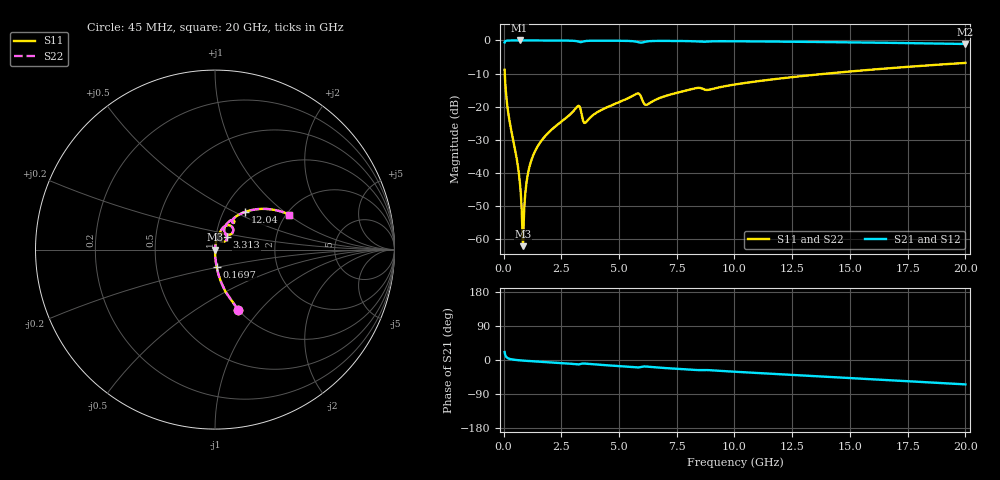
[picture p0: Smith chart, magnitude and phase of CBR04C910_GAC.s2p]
! S-parameter model data by Modelithics Inc.  support@modelithics.com 813-866-6335  Tampa FL USA
! S-Parameter data specifications:
! Substrate: 20-mil Rogers 4350B, substrate thickness, H=0.508mm, Dielectric constant, Er=3.75
! PCB Mounting Pad Footprint: Pad width, PadW=0.52mm , Pad length, PadL=0.52mm , Pad gap, PadG (edge-to-edge)=0.28mm , Reference planes=1.32mm apart
#  GHz  S  MA  R 50
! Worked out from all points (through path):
!   801 points, 45 MHz to 20 GHz, reference 50 ohm
!   highest |S21| = -0.01 dB at 693.5 MHz (marker M1); lowest = -1.1 dB at 20 GHz (marker M2)
!   group delay of S21, straight-line fit = 9.07 ps
!   lowest |S11| = -62.0 dB at 843.2 MHz (marker M3), VSWR 1.00, Z = 50.1 + j0.0259 ohm
!   |S11| at or under -10 dB: 53.06 MHz to 14 GHz (13.95 GHz wide, 198 % of centre)
!   |S22| runs from -62.0 to -6.8 dB; largest |S21 - S12| = 0
!   S11 on the Smith chart (normalised r, x): 45 MHz: 1.00, -0.77; 169.7 MHz: 1.00, -0.20; 3.313 GHz: 1.13, +0.16; 12.04 GHz: 1.26, +0.57; 20 GHz: 2.08, +1.02
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0.045  0.3605 -68.9  0.9326 21.0  0.9326 21.0  0.3605 -68.9
0.169719  0.09807 -84.5  0.9948 5.3  0.9948 5.3  0.09807 -84.5
0.568819  0.01656 -88.0  0.9992 -0.1  0.9992 -0.1  0.01656 -88.0
0.693538  0.007957 -86.0  0.9993 -0.8  0.9993 -0.8  0.007957 -86.0
0.768369  0.003679 -80.2  0.9993 -1.2  0.9993 -1.2  0.003679 -80.2
0.8432  0.000791 19.1  0.9992 -1.6  0.9992 -1.6  0.000791 19.1
0.918031  0.003922 76.7  0.9992 -1.9  0.9992 -1.9  0.003922 76.7
0.992862  0.007208 81.3  0.9991 -2.2  0.9991 -2.2  0.007208 81.3
1.092637  0.01132 83.0  0.9991 -2.7  0.9991 -2.7  0.01132 83.0
1.44185  0.02414 83.6  0.9987 -4.1  0.9987 -4.1  0.02414 83.6
2.115331  0.04629 81.7  0.9975 -6.6  0.9975 -6.6  0.04629 81.7
3.312631  0.09691 46.0  0.9435 -10.8  0.9435 -10.8  0.09691 46.0
3.387462  0.0746 39.5  0.9494 -9.5  0.9494 -9.5  0.0746 39.5
3.562069  0.05821 62.3  0.9804 -9.8  0.9804 -9.8  0.05821 62.3
5.757119  0.1573 59.2  0.9571 -19.5  0.9571 -19.5  0.1573 59.2
6.181163  0.1069 55.8  0.9635 -17.3  0.9635 -17.3  0.1069 55.8
6.704981  0.1332 66.6  0.983 -20.0  0.983 -20.0  0.1332 66.6
10.0225  0.2168 57.8  0.9713 -31.0  0.9713 -31.0  0.2168 57.8
12.04294  0.2686 51.4  0.9592 -37.8  0.9592 -37.8  0.2686 51.4
13.36496  0.3009 47.1  0.9496 -42.2  0.9496 -42.2  0.3009 47.1
16.68248  0.3804 36.2  0.9204 -53.2  0.9204 -53.2  0.3804 36.2
20  0.4583 25.1  0.8839 -64.3  0.8839 -64.3  0.4583 25.1
